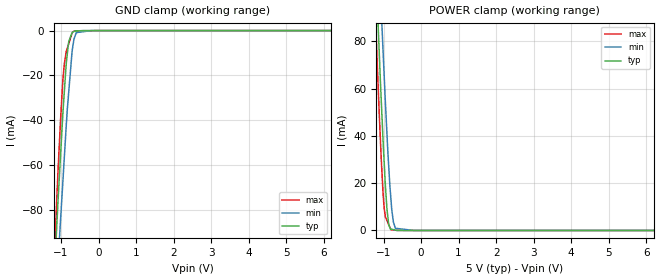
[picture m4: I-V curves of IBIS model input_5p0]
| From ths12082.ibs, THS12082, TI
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|   input_5p0 Model
[Model]   input_5p0
Model_type   Input
Vinl = 0.6
Vinh = 2.6
|   typ   min   max
|   (nom PVT)   (fast PVT)   (slow PVT)
C_comp   9.597e-13   9.523e-13   9.672e-13
| Where nom  PVT is Nominal Process, 5V, 27C
|   Fast PVT is Strong Process,  5.25V, -55C
|   Slow PVT is Weak Process,   4.75V, 125C
[Voltage Range]   5   4.75   5.25
|Ambient Temperature   25   125   -55
|Junction Temperature
[Temperature Range]   27   125   -55
[Power Clamp Reference]   5   4.75   5.25
[GND Clamp Reference]   0   0   0
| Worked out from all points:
|   GND clamp passes 1 mA (typ) near -0.71 V on its own axis
|   POWER clamp passes 1 mA (typ) near -0.83 V on its own axis
[GND Clamp]
|   Voltage   I(typ)   I(min)   I(max)
-5V       -1.642A    -1.561A    -1.765A
-1.306V   -152.3mA   -174.9mA   -149mA
-1.088V   -78.49mA   -106.4mA   -65.35mA
-1.036V   -62.48mA   -90.78mA   -47.43mA
-945mV    -35.31mA   -65.66mA   -20.86mA
-855mV    -13.59mA   -40.68mA   -8.966mA
-795mV    -4.964mA   -27.44mA   -5.832mA
-707.7mV  -970.8uA   -9.742mA   -1.275mA
-640.5mV  -218.9uA   -3.11mA    -155.4uA
-593.8mV  -169.5uA   -909.9uA   -144.1uA
-190mV    0A         -23.35nA   -46.1uA
10V       0A         0A         0A
[POWER Clamp]
|   Voltage   I(typ)   I(min)   I(max)
-5V       1.776A     1.782A     1.781A
-1.306V   150.2mA    188mA      126.8mA
-1.118V   76.66mA    115.1mA    50.84mA
-1.05V    51.11mA    89.17mA    26.83mA
-981.8mV  28.42mA    64.99mA    9.276mA
-910mV    9.312mA    41.17mA    4.23mA
-860mV    2.445mA    26.65mA    2.404mA
-803.3mV  599.5uA    13.29mA    330.8uA
-736.2mV  359.7uA    3.523mA    205.4uA
-684mV    172.7uA    932.3uA    107.5uA
-190mV    0A         0A         7.728uA
10V       0A         0A         0A
